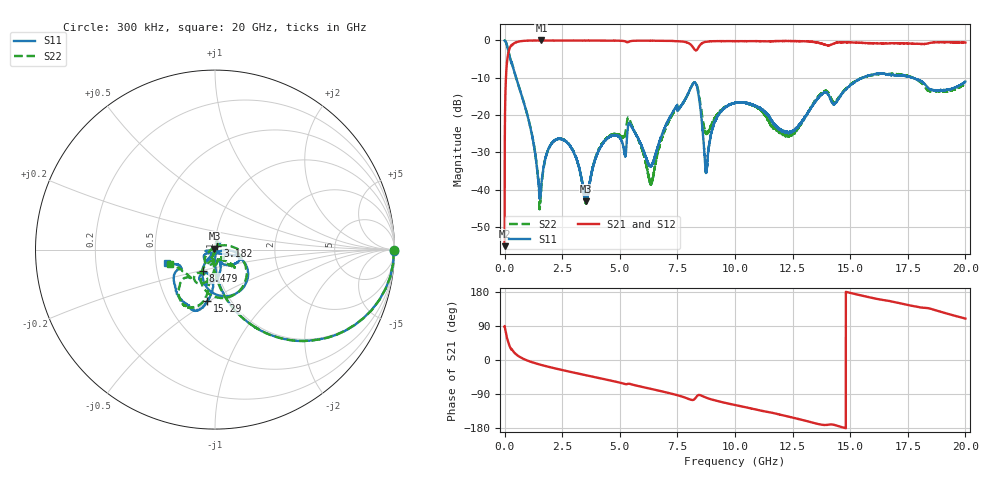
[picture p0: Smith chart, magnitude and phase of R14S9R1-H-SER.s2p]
!{R14S9R1}
!Johanson Technology Inc.
!www.johansontechnology.com
!Test Board Conditions:
!Substrate Type  RO4350B
!Substrate Thickness  20 mil
!Substrate Dk  3.66
!TL Type: GCPW
!TL Trace Width  36 mil
!TL Gap  12 mil
!Electrode orientation  Horizontal
!DUT TOPOLOGY	SERIES
!Mounting Pad LxW  26x36 mil
! Created Wed Nov 25 17:33:21 2020
! 2 Port Network Data from SP1.SP block
! freq  magS11  angS11  magS21  angS21  magS12  angS12  magS22  angS22
# khz S ma R 50
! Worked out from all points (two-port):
!   20001 points, 300 kHz to 20 GHz, reference 50 ohm
!   highest |S21| = -0.01 dB at 1.596 GHz (marker M1); lowest = -55.2 dB at 300 kHz (marker M2)
!   |S21| within 3 dB of the highest: 173.4 MHz to end of sweep
!   lowest |S11| = -43.2 dB at 3.529 GHz (marker M3), VSWR 1.01, Z = 49.7 + j0.603 ohm
!   |S11| at or under -10 dB: 500 MHz to 15.52 GHz (15.02 GHz wide, 188 % of centre); 15.52703 GHz to 15.52764 GHz (617.5 kHz wide, 0.00398 % of centre); 17.72 GHz to end of sweep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
!   |S22| runs from -45.3 to 0.0 dB; largest |S21 - S12| = 0.017
!   S11 on the Smith chart (normalised r, x): 300 kHz: open; 3.182 GHz: 1.03, +0.04; 8.479 GHz: 0.85, -0.20; 15.29 GHz: 0.78, -0.49; 20 GHz: 0.57, -0.10
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300  0.9968 -0.3  0.001744 88.6  0.001719 90.5  0.9967 -0.3
104300  0.856 -31.8  0.5134 58.1  0.5149 58.0  0.856 -31.8
206300  0.6358 -51.8  0.7676 37.9  0.7678 37.9  0.637 -51.8
1596300  0.01198 33.4  0.9993 -13.1  0.9983 -13.1  0.01078 112.3
2193300  0.04617 55.3  0.9977 -22.2  0.9968 -22.2  0.04606 78.6
3182300  0.02227 54.0  0.9973 -35.6  0.9974 -35.6  0.02227 54.8
3334300  0.01419 62.7  0.9969 -37.6  0.997 -37.6  0.01397 42.2
3529300  0.006948 119.1  0.9969 -40.2  0.997 -40.2  0.006596 -21.5
4215300  0.03967 -168.9  0.9954 -49.2  0.9953 -49.2  0.04079 -108.9
5383300  0.07623 -130.5  0.9561 -62.6  0.9561 -62.7  0.09333 -121.0
6325300  0.02113 -94.8  0.9932 -75.8  0.9929 -75.9  0.01185 129.3
6667300  0.03914 -36.4  0.9932 -80.6  0.9923 -80.6  0.03331 41.3
8185300  0.2643 -53.7  0.8026 -105.4  0.8012 -105.3  0.2657 -58.3
8479300  0.1362 -120.3  0.8637 -92.6  0.8634 -92.5  0.1536 -119.7
8757300  0.01745 -49.1  0.9614 -99.6  0.9613 -99.6  0.05623 -86.1
9172300  0.08676 -3.5  0.9785 -107.2  0.9789 -107.2  0.09495 -44.6
1.00003e7  0.1452 -17.9  0.979 -118.7  0.9782 -118.8  0.1453 -42.0
1.22693e7  0.05912 -68.3  0.9833 -148.7  0.9839 -148.6  0.05383 -55.8
1.33343e7  0.1298 -77.8  0.9605 -164.7  0.9618 -164.7  0.1322 -94.8
1.52883e7  0.2885 -98.6  0.9349 173.1  0.939 172.6  0.2919 -101.9
1.66673e7  0.3443 -114.9  0.9139 156.0  0.907 155.5  0.3541 -117.7
2e7  0.2802 -164.1  0.9363 109.3  0.9344 109.6  0.2657 -162.9
